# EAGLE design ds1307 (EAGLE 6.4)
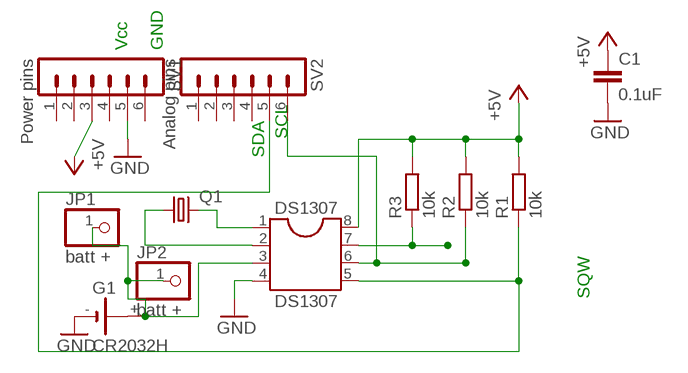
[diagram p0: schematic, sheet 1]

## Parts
C1  0.1uF  C-EU050-024X044  [C050-024X044]
DS1307  DS1307  DIL8  [DIL08]
G1  CR2032H  [CR2032H]
JP1  batt +  PINHD-1X1  [1X01]
JP2  batt +  PINHD-1X1  [1X01]
Q1  CRYSTALTC38H  [TC38H]
R1  10k  R-EU_0207/7  [0207/7]
R2  10k  R-EU_0207/7  [0207/7]
R3  10k  R-EU_0207/7  [0207/7]
SV1  Power pins  MA06-1  [MA06-1]
SV2  Analog pins  MA06-1  [MA06-1]

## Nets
+5V: C1.1 DS1307.8 R1.2 R2.2 R3.2 SV1.3
GND: C1.2 DS1307.4 G1.- SV1.5
N$2: DS1307.7 R3.1
N$4: DS1307.5 R1.1 SV2.5
N$5: DS1307.3 G1.+ JP1.1 JP2.1
N$7: DS1307.1 Q1.2
N$8: DS1307.2 Q1.1
N$9: DS1307.6 R2.1 SV2.6
Unconnected: G1.+@1(+) SV1.1 SV1.2 SV1.4 SV1.6 SV2.1 SV2.2 SV2.3 SV2.4

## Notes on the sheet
- Vcc | GND
- SDA
- SCL
- SQW

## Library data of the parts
C1 = rcl:C-EU: CAPACITOR, European symbol
DS1307 = ic-package:DIL8: Dual In Line / Socket
G1 = battery:CR2032H: LI BATTERY Varta
JP1 JP2 = pinhead:PINHD-1X1: PIN HEADER
Q1 = crystal:CRYSTAL: CRYSTAL
R1-R3 = rcl:R-EU_: RESISTOR, European symbol
SV1 SV2 = con-lstb:MA06-1: PIN HEADER; OC_FARNELL: unknown; OC_NEWARK: unknown

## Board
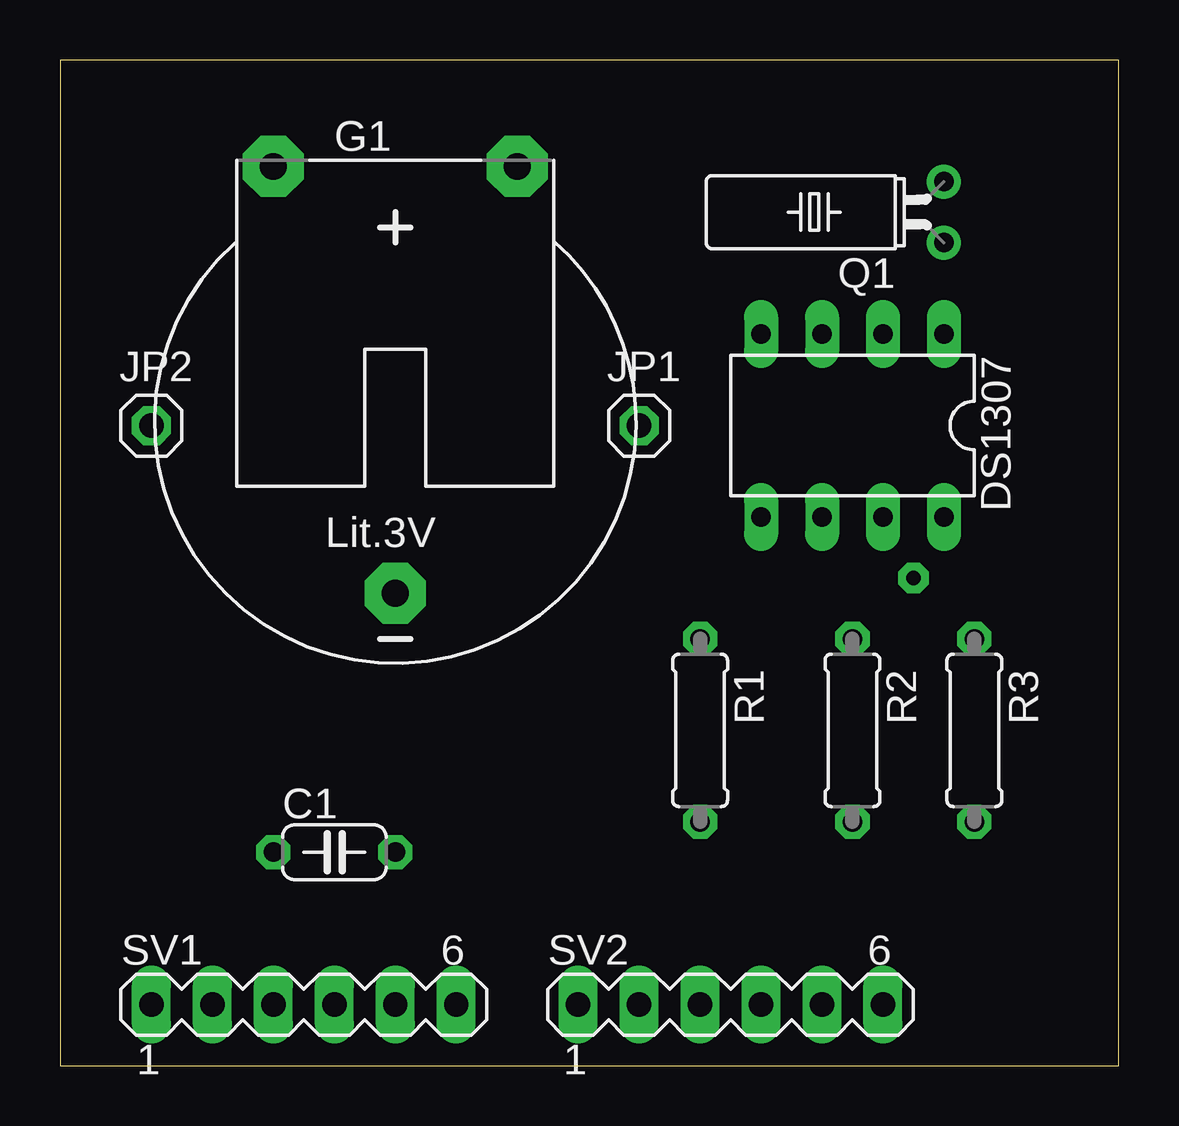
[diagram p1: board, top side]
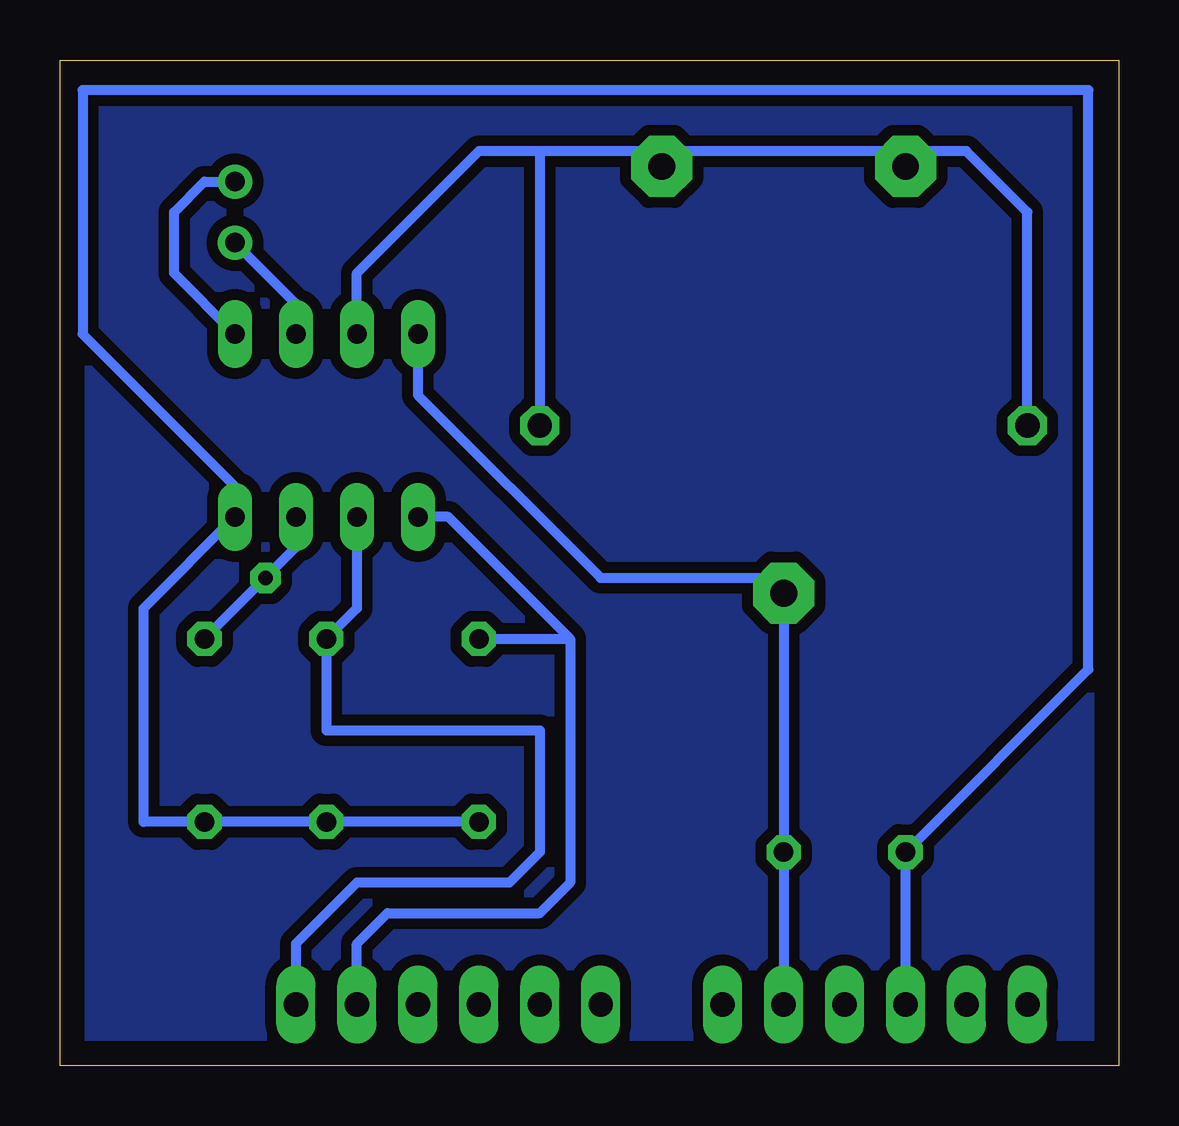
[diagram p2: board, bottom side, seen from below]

Size 44.12 x 41.9 mm. Coordinates in mm from the lower left corner, seen from the top.
Outline: 0,0 44.12,0 44.12,41.9 0,41.9 0,0
Copper layers (1*16): Top 0.035mm / dielectric 1.5mm / Bottom 0.035mm
Design rules "default *": minimum track width 10mil, minimum drill 24mil, track to track 18mil, track to pad 18mil, pad to pad 18mil, via to via 18mil, smd to smd 8mil, copper to edge 40mil, drill to drill 18mil, minimum pad ring 12mil, minimum via ring 12mil, stop-mask expansion 4mil, vias tented up to drill 0mil, thermal gap 10mil

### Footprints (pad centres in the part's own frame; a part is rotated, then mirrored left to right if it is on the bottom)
C050-024X044 = drill 0.813 octagon: 1 -2.54,0; 2 2.54,0
DIL08 = drill 0.813 long: 1 -3.81,-3.81; 2 -1.27,-3.81; 3 1.27,-3.81; 4 3.81,-3.81; 5 3.81,3.81; 6 1.27,3.81; 7 -1.27,3.81; 8 -3.81,3.81
CR2032H = drill 1.118 pad 2.54 octagon: + 5.08,10.795; +@1 -5.08,10.795; - 0,-6.985
1X01 = drill 1.016 octagon: 1 0,0
TC38H = drill 0.813: 1 -1.27,0; 2 1.27,0
0207/7 = drill 0.813 octagon: 1 -3.81,0; 2 3.81,0
MA06-1 = drill 1.016 long: 1 -6.35,0; 2 -3.81,0; 3 -1.27,0; 4 1.27,0; 5 3.81,0; 6 6.35,0

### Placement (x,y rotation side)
C1  11.43,8.89 0 top
DS1307  33.02,26.67 180 top
G1  13.97,26.67 0 top
JP1  24.13,26.67 0 top
JP2  3.81,26.67 0 top
Q1  36.83,35.56 90 top
R1  26.67,13.97 270 top
R2  33.02,13.97 270 top
R3  38.1,13.97 270 top
SV1  10.16,2.54 0 top
SV2  27.94,2.54 0 top

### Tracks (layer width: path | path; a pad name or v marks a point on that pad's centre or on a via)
+5V
  Bottom 0.406: SV1.3 C1.1 1.27,16.51 1.27,40.64 43.18,40.64 43.18,30.48 36.83,24.13 DS1307.8 40.64,19.05 40.64,10.16 R3.2 R2.2 R1.2
GND
  Bottom 0.406: DS1307.4 29.21,27.94 21.59,20.32 13.97,20.32 G1.- C1.2 SV1.5
N$2  (via drill 0.6 pad 1.27)
  Bottom 0.406: DS1307.7 34.29,21.59 v35.56,20.32 R3.1
N$3
  pour Bottom: 0,41.91 44.45,41.91 44.45,0 0,0
N$4
  Bottom 0.406: SV2.5 31.75,5.08 30.48,6.35 24.13,6.35 22.86,7.62 22.86,17.78 | R1.1 22.86,17.78 | 22.86,17.78 27.94,22.86 DS1307.5
N$5
  Bottom 0.406: DS1307.3 31.75,33.02 26.67,38.1 24.13,38.1 | 24.13,38.1 JP1.1 | JP2.1 3.81,35.56 6.35,38.1 19.05,38.1 | 19.05,38.1 24.13,38.1 | G1.+ 19.05,38.1
N$7
  Bottom 0.406: DS1307.1 39.37,33.02 39.37,35.56 38.1,36.83 Q1.2
N$8
  Bottom 0.406: Q1.1 34.29,31.75 DS1307.2
N$9
  Bottom 0.406: SV2.6 34.29,5.08 31.75,7.62 25.4,7.62 24.13,8.89 24.13,13.97 33.02,13.97 R2.1 31.75,19.05 DS1307.6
